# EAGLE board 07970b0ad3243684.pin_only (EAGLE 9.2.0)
REV: B

Size 20.32 x 13.97 mm. Coordinates in mm from the lower left corner, seen from the top.
Outline: 20.32,11.43 20.32,2.54 arc-90 17.78,0 2.54,0 arc-90 0,2.54 0,11.43 arc-90 2.54,13.97 17.78,13.97 arc-90 20.32,11.43
Copper layers (1*16): Top 0.035mm / dielectric 1.5mm / Bottom 0.035mm
Design rules "adafruit": minimum track width 8mil, minimum drill 15.5mil, track to track 8mil, track to pad 8mil, pad to pad 8mil, via to via 8mil, smd to smd 8mil, copper to edge 10mil, drill to drill 8mil, minimum pad ring 10mil, minimum via ring 8mil, stop-mask expansion 2mil, vias tented up to drill 20mil, thermal gap 10mil

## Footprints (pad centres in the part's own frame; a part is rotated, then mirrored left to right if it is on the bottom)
FIDUCIAL_1MM = smd 1 x 1: 1 0,0
1X08_ROUND_76 = drill 1 pad 1.93: 1 -8.89,0; 2 -6.35,0; 3 -3.81,0; 4 -1.27,0; 5 1.27,0; 6 3.81,0; 7 6.35,0; 8 8.89,0
0603-NO = smd 1.075 x 1: 1 -0.85,0; 2 0.85,0
MOUNTINGHOLE_2.5_PLATED = drill 2.5 pad 3.2: P$1 0,0
USB_C_CUSB31-CFM2AX-01-X = smd 0.575 x 1.15: A1B12 -3.2,7.355; A4B9 -2.4,7.355; B1A12 3.2,7.355; B4A9 2.4,7.355 | smd 0.275 x 1.15: A5 -1.25,7.355; A6 -0.25,7.355; A7 0.25,7.355; A8 1.25,7.355; B5 1.75,7.355; B6 0.75,7.355; B7 -0.75,7.355; B8 -1.75,7.355 | drill 0.6 pad 1 long: M1 -4.32,6.78; M2 4.32,6.78; M3 -4.32,2.6; M4 4.32,2.6 | hole 0.65: 2.89,6.28; -2.89,6.28

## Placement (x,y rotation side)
FID1  FIDUCIAL_1MM  [FIDUCIAL_1MM]  12.7,9.4 180 top
FID2  FIDUCIAL_1MM  [FIDUCIAL_1MM]  7.62,12.57 180 top
JP1  [1X08_ROUND_76]  10.16,2.54 180 top
R1  5.1K  [0603-NO]  2.03,5.84 0 top
R2  5.1K  [0603-NO]  2.03,7.62 0 top
U$1  MOUNTINGHOLE2.5  [MOUNTINGHOLE_2.5_PLATED]  17.78,11.43 180 top
U$2  MOUNTINGHOLE2.5  [MOUNTINGHOLE_2.5_PLATED]  2.54,11.43 180 top
U$3  [ADAFRUIT_2.5MM]  18.8,9.14 180 top
U$8  [PCBFEAT-REV-040]  1.63,4.88 180 bottom
X1  [USB_C_CUSB31-CFM2AX-01-X]  10.16,13.97 180 top

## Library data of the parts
FID1 FID2 U$1 U$2 = microbuilder; BOM: EXCLUDE
JP1 R1 R2 U$3 U$8 X1 = microbuilder

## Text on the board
tPlace: USB C | SBU1 | D- | SBU2 | GND | CC2 | D+ | CC1 | VBUS
bPlace: adafruit! | downstream / (periph.) / USB C Breakout

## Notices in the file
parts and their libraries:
microbuilder: This work is placed in the public domain, and may be freely used for commercial and non-commercial work with the following conditions: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
